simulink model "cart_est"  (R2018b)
settings: Solver=ode4  StartTime=0.0  StopTime=10.0  FixedStep=1e-3  RelTol=1e-3
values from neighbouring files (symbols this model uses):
  k_1 = 1 / m    [mainSkript_estimaceVozik.m]    (also in mainSkript_odhadKyvadlaZvlast.m = params.k_1; mainSkript_kyvadlaNajednouOdhad.m = params.k_1; mainSkript_modifikaceVozik.m = 0.695894224078)
  kn = bn_0 / m    [mainSkript_estimaceVozik.m]    (also in mainSkript_modifikaceVozik.m)
  kp = bp_0 / m    [mainSkript_estimaceVozik.m]    (also in mainSkript_modifikaceVozik.m = 1.28051496173)
  v_0 = v(n_start)    [mainSkript_estimaceVozik.m]    (also in mainSkript_modifikaceVozik.m = v(1))
  x_0 = x(n_start)    [mainSkript_estimaceVozik.m]    (also in mainSkript_modifikaceVozik.m = x(1))
libraries: simulink x1

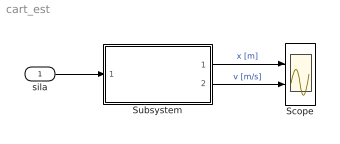
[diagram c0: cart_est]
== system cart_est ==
  sila : Inport
  Scope : Scope  NumInputPorts=2
  Subsystem : Subsystem
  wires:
  Subsystem/1(x) -> Scope/1  "x [m]"
  sila/1 -> Subsystem/1(sila [N])
  Subsystem/2(v) -> Scope/2  "v [m/s]"

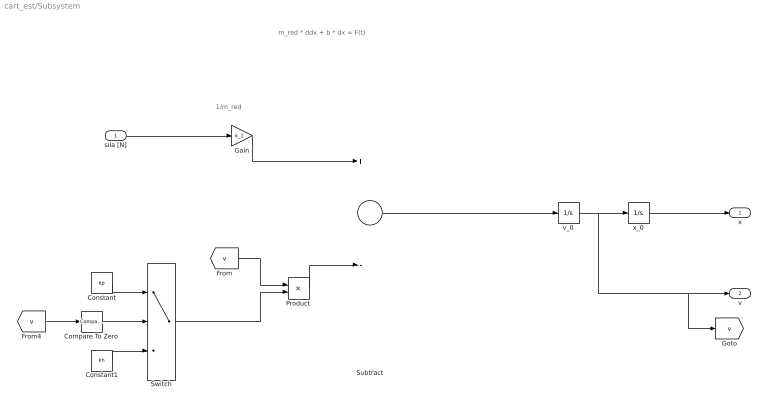
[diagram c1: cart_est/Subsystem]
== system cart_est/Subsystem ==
  note: 1/m_red
  note: m_red * ddx + b * dx = F(t)
  sila [N] : Inport
  Compare To Zero : simulink/Logic and Bit Operations/Compare To Zero  relop=>  OutDataTypeStr=boolean
  Constant : Constant  Value=kp
  Constant1 : Constant  Value=kn
  Gain : Gain  Gain=k_1
  Product : Product
  Subtract : Sum  Inputs=+-
  Switch : Switch  Criteria=u2 > Threshold
  v_0 : Integrator  InitialCondition=v_0
  x_0 : Integrator  InitialCondition=x_0
  x : Outport
  v : Outport  Port=2
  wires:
  Product/1 -> Subtract/2
  x_0/1 -> x/1
  [v] -> Product/1
  Constant1/1 -> Switch/3
  Compare To Zero/1 -> Switch/2
  [v] -> Compare To Zero/1
  Constant/1 -> Switch/1
  Switch/1 -> Product/2
  v_0/1 -> v/1, [v], x_0/1
  sila [N]/1 -> Gain/1
  Subtract/1 -> v_0/1
  Gain/1 -> Subtract/1
